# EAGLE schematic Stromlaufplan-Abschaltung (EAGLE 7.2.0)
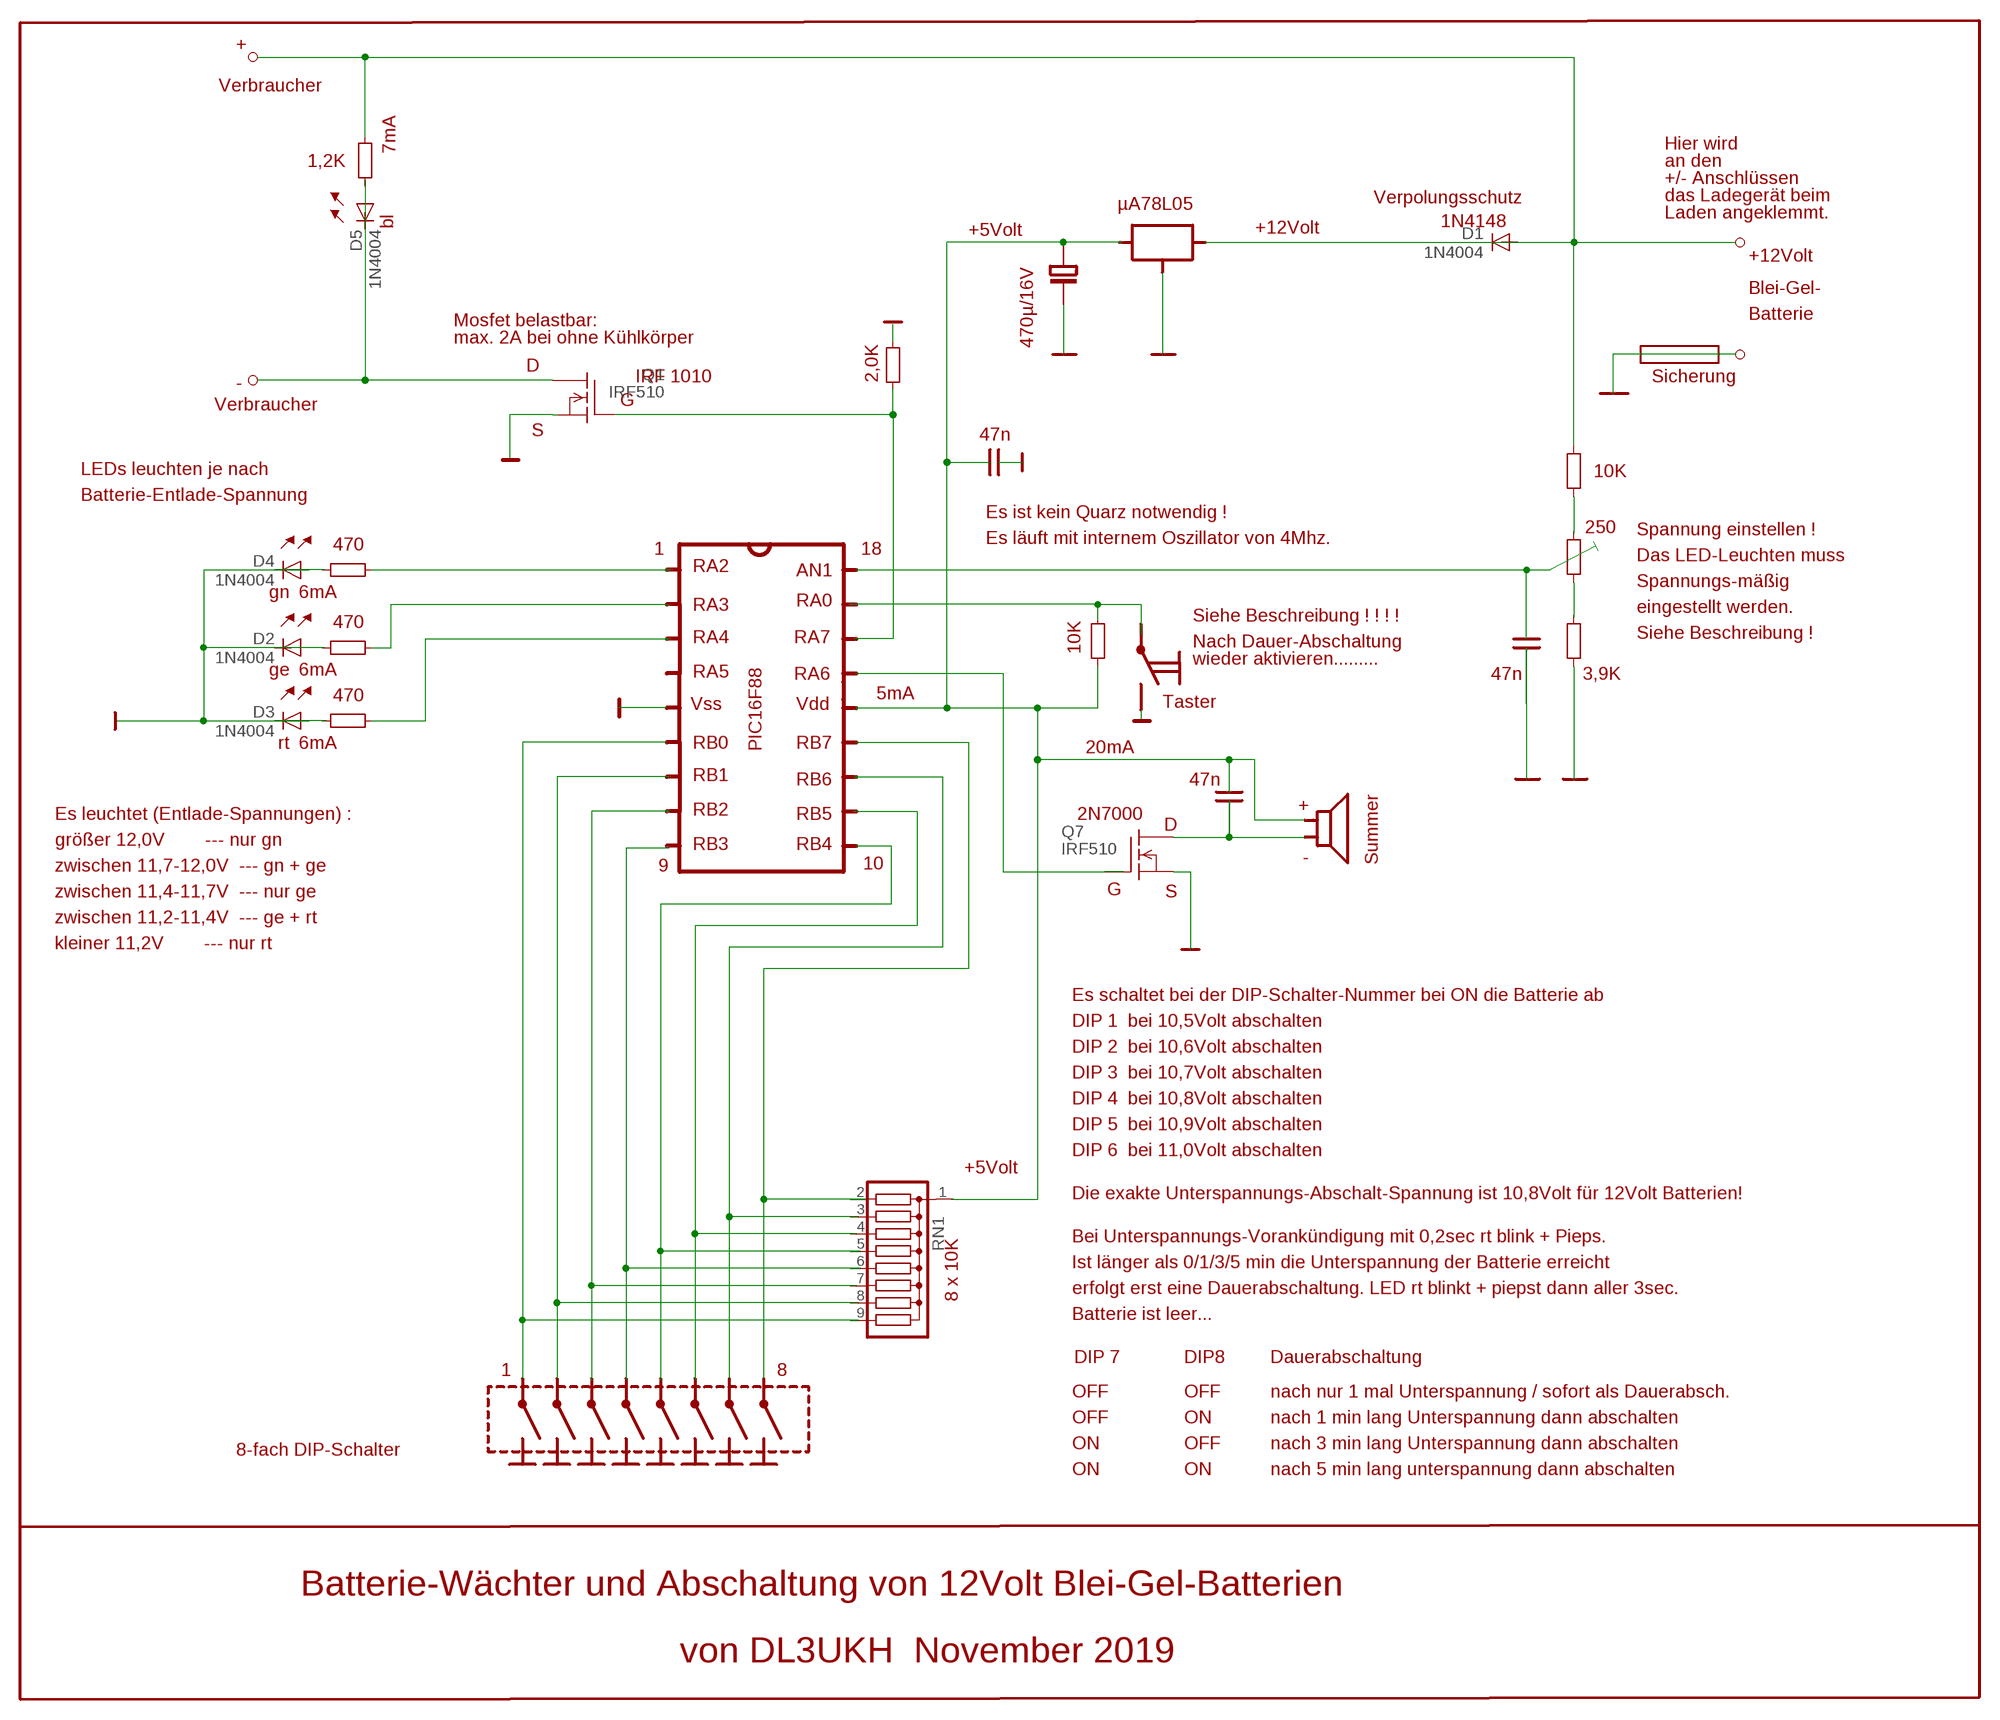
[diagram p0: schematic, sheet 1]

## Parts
D1  1N4004  [DO41-10]
D2  1N4004  [DO41-10]
D3  1N4004  [DO41-10]
D4  1N4004  [DO41-10]
D5  1N4004  [DO41-10]
Q1  IRF510  [TO220]
Q7  IRF510  [TO220]
RN1  G08R  [SIL9]

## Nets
N$8: RN1.9
N$9: RN1.8
N$10: RN1.7
N$11: RN1.6
N$12: RN1.5
N$13: RN1.4
N$14: RN1.3
N$15: RN1.2
N$17: D2.C
N$19: D2.A D3.A D4.A
N$20: Q1.3(S)
N$21: D3.C
N$25: Q7.3(S)
N$26: Q7.2(D)
N$28: D4.C
N$31: D5.A D5.C Q1.2(D)
N$32: RN1.1
N$36: Q1.1(G)
N$38: D1.A D1.C
N$69: Q7.1(G)

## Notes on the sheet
- +
- Verbraucher
- 7mA
- 1,2K | Hier wird
- an den
- +/- Anschlüssen
- Verpolungsschutz | das Ladegerät beim
- bl | µA78L05
- +5Volt | Laden angeklemmt.
- 1N4148
- +12Volt
- +12Volt
- Blei-Gel-
- Batterie
- Mosfet belastbar:
- max. 2A bei ohne Kühlkörper | 470µ/16V
- D
- IRF 1010 | 2,0K | Sicherung
- -
- Verbraucher
- G
- S | 47n
- LEDs leuchten je nach | 10K
- Batterie-Entlade-Spannung
- Es ist kein Quarz notwendig !
- 250 | Spannung einstellen !
- Es läuft mit internem Oszillator von 4Mhz.
- 470 | 1 | 18
- Das LED-Leuchten muss
- RA2 | AN1
- gn | 6mA | Spannungs-mäßig
- RA3 | RA0
- eingestellt werden.
- Siehe Beschreibung ! ! ! !
- 470
- RA4 | RA7 | Siehe Beschreibung !
- Nach Dauer-Abschaltung
- 10K
- ge | 6mA | wieder aktivieren......... | 47n
- RA5 | RA6 | 3,9K
- 5mA
- 470
- Vss | Vdd | Taster
- rt | 6mA | 20mA
- RB0 | PIC16F88 | RB7
- 47n
- RB1 | RB6
- + | Summer
- Es leuchtet (Entlade-Spannungen) : | RB2 | RB5 | 2N7000
- D
- größer 12,0V        --- nur gn | RB3 | RB4 | -
- zwischen 11,7-12,0V  --- gn + ge | 9 | 10
- zwischen 11,4-11,7V  --- nur ge | G | S
- zwischen 11,2-11,4V  --- ge + rt
- kleiner 11,2V        --- nur rt
- Es schaltet bei der DIP-Schalter-Nummer bei ON die Batterie ab
- DIP 1  bei 10,5Volt abschalten
- DIP 2  bei 10,6Volt abschalten
- DIP 3  bei 10,7Volt abschalten
- DIP 4  bei 10,8Volt abschalten
- DIP 5  bei 10,9Volt abschalten
- +5Volt | DIP 6  bei 11,0Volt abschalten
- Die exakte Unterspannungs-Abschalt-Spannung ist 10,8Volt für 12Volt Batterien!
- 8 x 10K | Bei Unterspannungs-Vorankündigung mit 0,2sec rt blink + Pieps.
- Ist länger als 0/1/3/5 min die Unterspannung der Batterie erreicht
- erfolgt erst eine Dauerabschaltung. LED rt blinkt + piepst dann aller 3sec.
- Batterie ist leer...
- DIP 7 | DIP8 | Dauerabschaltung
- 1 | 8
- OFF | OFF | nach nur 1 mal Unterspannung / sofort als Dauerabsch.
- OFF | ON | nach 1 min lang Unterspannung dann abschalten
- ON | OFF | nach 3 min lang Unterspannung dann abschalten
- 8-fach DIP-Schalter
- ON | ON | nach 5 min lang unterspannung dann abschalten
- Batterie-Wächter und Abschaltung von 12Volt Blei-Gel-Batterien
- von DL3UKH  November 2019

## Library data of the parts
D1-D5 = diode:1N4004: DIODE
Q1 Q7 = transistor-fet:IRF510: N-Channel Enhancement MOSFET (HEXFET); 100V; 5,6A; 0,54Ohm
RN1 = resistor-sil:G08R: SIL RESISTOR; OC_FARNELL: unknown; OC_NEWARK: unknown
